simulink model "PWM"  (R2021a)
settings: Solver=FixedStepDiscrete  StartTime=0.0  StopTime=Inf  RelTol=1e-3  EnableMultiTasking=on
undefined symbols (not defined in the file or in its folder): A, ADCIN0, ADCIN1, ADCINA0, ADCINB0, bit, Compare, conversion, Count, DCAEVT1, DCAEVT1FILT, Digital, Down, edge, ended, Event, falling, Filtered, GPTRIP1SEL, GPTRIP2SEL, input, Module, of, resolution, rising, Single, start, the, Trip, TZ1, TZ2, Up, version, Zone
libraries: c2802xlib x9, c280xlib x2

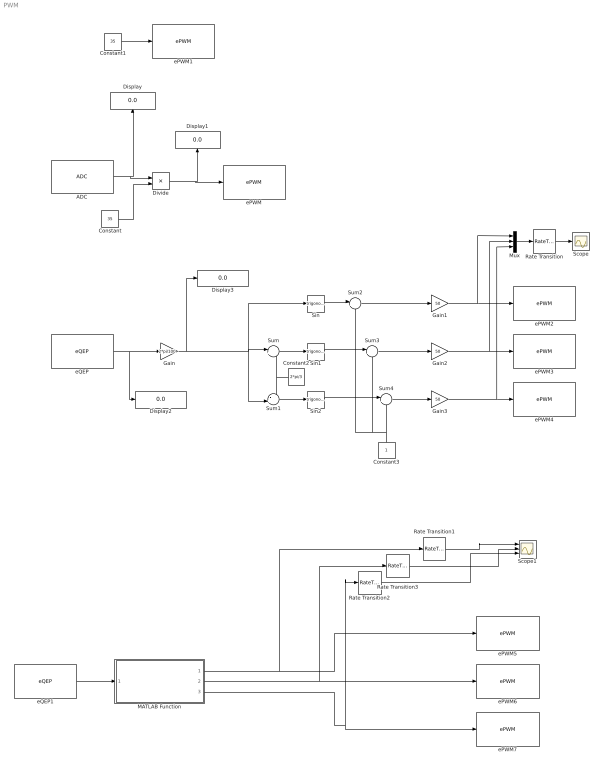
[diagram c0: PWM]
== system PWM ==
  ADC : c2802xlib/ADC  Commented=on  blkParamProc=C2000  ADCModule=1  samplingMode=Single sample mode  ADCResolution=12-bit (Single-ended input)  useSOC1=SOC0  useSOC2=SOC0_SOC1  SOCAcquisitionWindow=7  SOCTriggerSource=CPU0_TINT0n  SOCInterruptTrigger=No ADCINT  Ts=0.001  dType=uint16  postInterrupt=off  interruptSel=ADCINT1  ADCINTContinuous=off  endma=off  chdma=1  conv1=ADCINA6  conv2=ADCINA0 and ADCINB0  conv1_Type4=ADCIN0  conv2_Type4=ADCIN0 and ADCIN1
  Constant : Constant  Commented=on  Value=35
  Constant1 : Constant  Commented=on  Value=35
  Constant2 : Constant  Commented=on  Value=2*pi/3
  Constant3 : Constant  Commented=on
  Display{,1..3} (4 alike) : Display
  Divide : Product  Commented=on  Inputs=*/
  Gain : Gain  Commented=on  Gain=2*pi/100
  Gain1 : Gain  Commented=on  Gain=50
  Gain2 : Gain  Commented=on  Gain=50
  Gain3 : Gain  Commented=on  Gain=50
  MATLAB Function : MATLAB Function  TreatAsAtomicUnit=on
  Mux : Mux  Commented=on  Inputs=3
  Rate Transition : RateTransition  Commented=on
  Rate Transition1 : RateTransition
  Rate Transition2 : RateTransition
  Rate Transition3 : RateTransition
  Scope : Scope
  Scope1 : Scope  NumInputPorts=3
  Sin : Trigonometry  Commented=on
  Sin1 : Trigonometry  Commented=on
  Sin2 : Trigonometry  Commented=on
  Sum{,2..4} (4 alike) : Sum  Commented=on  Inputs=|++
  Sum1 : Sum  Commented=on  Inputs=-+|
  ePWM : c2802xlib/ePWM  Commented=on  PwmType=C2000  useModule=ePWM4  ePWMxLINKTBPRD=Not Linked  periodUnits=Seconds  timerSource=Specify via dialog  timerPeriod_clk=64000  timerPeriod_sec=0.0001  tbshadow=Counter equals to zero  countingMode=Up-Down  phaseActiveEnable=Disable  phaseDirection=Count down after sync  phaseActive=0  synchronizationEnable=off  dcaevt1Sync=off  dcbevt1Sync=off  synchronizationOption=Disable  perSynchronizationOption=Counter equals to period (CTR=PRD)  clockPrescale=1  HSclockPrescale=1  enswap=off  ePWMxAStatus=on  ePWMxAactionLogic1=Do nothing  ePWMxAactionLogic2=Do nothing  ePWMxAactionLogic3=Set  ePWMxAactionLogic4=Clear  ePWMxAactionLogic5=Do nothing  ePWMxAactionLogic6=Do nothing  ePWMxACSFenable=off  ePWMxACSFvalue=Forcing disable  ePWMxASFreload=Zero  ePWMxBStatus=off  ePWMxBactionLogic1=Set  ePWMxBactionLogic2=Clear  ePWMxBactionLogic3=Do nothing  ePWMxBactionLogic4=Do nothing  ePWMxBactionLogic5=Clear  ePWMxBactionLogic6=Set  ePWMxBCSFenable=off  ePWMxBCSFvalue=Forcing disable  ePWMxBSFreload=Zero  ePWNxBOutWay=off  ePWMxLINKCMPA=Not Linked  CMPAUnits=Percentages  CMPASource=Input port  CMPAValue_per=0  CMPAValue_clk=32000  enCMPAshadow=Counter equals to zero (CTR=Zero)  ePWMxLINKCMPB=Not Linked  CMPBUnits=Clock cycles  CMPBSource=Specify via dialog  CMPBValue_per=50  CMPBValue_clk=32000  enCMPBshadow=Counter equals to zero (CTR=Zero)  ePWMxLINKCMPC=Not Linked  CMPCUnits=Clock cycles  CMPCSource=Specify via dialog  CMPCValue_per=50  CMPCValue_clk=32000  enCMPCshadow=Counter equals to zero (CTR=Zero)  ePWMxLINKCMPD=Not Linked  CMPDUnits=Clock cycles  CMPDSource=Specify via dialog  CMPDValue_per=50  CMPDValue_clk=32000  enCMPDshadow=Counter equals to zero (CTR=Zero)  enableDBePWMxA=off  enableDBePWMxB=off  enhalfcycle=off  DBpolarity=Active high (AH)  DBedgeDelay=Positive  DBSource_ePWMxA=ePWMxA  DBSource_ePWMxB=ePWMxA  DBPeriodUnits=Clock cycles  DBperiodSource=Specify via dialog  REDperiod=0  FEDperiod=0  REDperiod_sec=0  FEDperiod_sec=0  LoadModeDBRED=Immediate without using shadow  LoadModeDBFED=Immediate without using shadow  adcstartModuleA=off  adcrequestEventA=First event  adcstartEventA=Counter equals to zero (CTR=Zero)  adcstartEventA_type2=Digital Compare Module A Event 1 start of conversion (DCAEVT1.soc)  adcstartModuleB=off  adcrequestEventB=First event  adcstartEventB=Counter equals to zero (CTR=Zero)  adcstartEventB_type2=Counter equals to zero (CTR=Zero)  intEn=off  intPrd=First event  intSel=Counter equals to zero (CTR=Zero)  intSel_type2=Counter equals to zero (CTR=Zero)  hrpe=off  enHRPWM=off  HRPWM_LoadMode=Counter equals to period (CTR=PRD)  HRPWM_CTLMode=Duty or Period control mode  HRPWM_EDGMode=Both edge  hrpeb=off  enHRPWMB=off  HRPWM_LoadModeB=Counter equals to zero (CTR=ZERO)  HRPWM_CTLModeB=Duty or Period control mode  HRPWM_EDGModeB=Both edge  enHRDBRED=off  enHRDBFED=off  enSFO=on  enautoconv=on  chopperEnable=off  chopperFrequency=1  chopperFirstwidth=1  chopperDuty=12.5%  tripZonesource=Specify via dialog  tzselOSHT1=off  tzselOSHT2=off  tzselOSHT3=off  tzselOSHDCAEV1=off  tzselOSHDCBEV1=off  tzselCBC1=off  tzselCBC2=off  tzselCBC3=off  tzselCBCDCAEV2=off  tzselCBCDCBEV2=off  tzselOSHT4=off  tzselOSHT5=off  tzselOSHT6=off  tzselCBC4=off  tzselCBC5=off  tzselCBC6=off  enTzOstIntr=off  enTzCbcIntr=off  enTzDCAEVT1Intr=off  enTzDCAEVT2Intr=off  enTzDCBEVT1Intr=off  enTzDCBEVT2Intr=off  ePWMxAforced=No action  ePWMxBforced=No action  DCAEVT1forced=No action  DCBEVT1forced=No action  DCAEVT2forced=No action  DCBEVT2forced=No action  dcah=Trip Zone 1 input (TZ1)  dcal=Trip Zone 1 input (TZ1)  dcbh=Trip Zone 1 input (TZ1)  dcbl=Trip Zone 1 input (TZ1)  dcah_type2=GPTRIP1SEL/(TZ1)  dcal_type2=GPTRIP2SEL/(TZ2)  dcbh_type2=GPTRIP1SEL/(TZ1)  dcbl_type2=GPTRIP2SEL/(TZ2)  gendcaevt1=Event disabled  gendcaevt2=Event disabled  gendcbevt1=Event disabled  gendcbevt2=Event disabled  dcaevt1src=DCAEVT1 with sync  dcaevt2src=DCAEVT2 with sync  dcbevt1src=DCBEVT1 with sync  dcbevt2src=DCBEVT2 with sync  pulsesel=Counter equals to zero (CTR=Zero)  blankinv=off  blankoffset=0  blankwidth=0  evsrcsel=Filtered version of DCAEVT1 (DCAEVT1FILT)  encape=off
  ePWM1 : c2802xlib/ePWM  Commented=on  PwmType=C2000  useModule=ePWM4  ePWMxLINKTBPRD=Not Linked  periodUnits=Seconds  timerSource=Specify via dialog  timerPeriod_clk=64000  timerPeriod_sec=0.0001  tbshadow=Counter equals to zero  countingMode=Up-Down  phaseActiveEnable=Disable  phaseDirection=Count down after sync  phaseActive=0  synchronizationEnable=off  dcaevt1Sync=off  dcbevt1Sync=off  synchronizationOption=Disable  perSynchronizationOption=Counter equals to period (CTR=PRD)  clockPrescale=1  HSclockPrescale=1  enswap=off  ePWMxAStatus=on  ePWMxAactionLogic1=Do nothing  ePWMxAactionLogic2=Do nothing  ePWMxAactionLogic3=Set  ePWMxAactionLogic4=Clear  ePWMxAactionLogic5=Do nothing  ePWMxAactionLogic6=Do nothing  ePWMxACSFenable=off  ePWMxACSFvalue=Forcing disable  ePWMxASFreload=Zero  ePWMxBStatus=off  ePWMxBactionLogic1=Set  ePWMxBactionLogic2=Clear  ePWMxBactionLogic3=Do nothing  ePWMxBactionLogic4=Do nothing  ePWMxBactionLogic5=Clear  ePWMxBactionLogic6=Set  ePWMxBCSFenable=off  ePWMxBCSFvalue=Forcing disable  ePWMxBSFreload=Zero  ePWNxBOutWay=off  ePWMxLINKCMPA=Not Linked  CMPAUnits=Percentages  CMPASource=Input port  CMPAValue_per=0  CMPAValue_clk=32000  enCMPAshadow=Counter equals to zero (CTR=Zero)  ePWMxLINKCMPB=Not Linked  CMPBUnits=Clock cycles  CMPBSource=Specify via dialog  CMPBValue_per=50  CMPBValue_clk=32000  enCMPBshadow=Counter equals to zero (CTR=Zero)  ePWMxLINKCMPC=Not Linked  CMPCUnits=Clock cycles  CMPCSource=Specify via dialog  CMPCValue_per=50  CMPCValue_clk=32000  enCMPCshadow=Counter equals to zero (CTR=Zero)  ePWMxLINKCMPD=Not Linked  CMPDUnits=Clock cycles  CMPDSource=Specify via dialog  CMPDValue_per=50  CMPDValue_clk=32000  enCMPDshadow=Counter equals to zero (CTR=Zero)  enableDBePWMxA=off  enableDBePWMxB=off  enhalfcycle=off  DBpolarity=Active high (AH)  DBedgeDelay=Positive  DBSource_ePWMxA=ePWMxA  DBSource_ePWMxB=ePWMxA  DBPeriodUnits=Clock cycles  DBperiodSource=Specify via dialog  REDperiod=0  FEDperiod=0  REDperiod_sec=0  FEDperiod_sec=0  LoadModeDBRED=Immediate without using shadow  LoadModeDBFED=Immediate without using shadow  adcstartModuleA=off  adcrequestEventA=First event  adcstartEventA=Counter equals to zero (CTR=Zero)  adcstartEventA_type2=Digital Compare Module A Event 1 start of conversion (DCAEVT1.soc)  adcstartModuleB=off  adcrequestEventB=First event  adcstartEventB=Counter equals to zero (CTR=Zero)  adcstartEventB_type2=Counter equals to zero (CTR=Zero)  intEn=off  intPrd=First event  intSel=Counter equals to zero (CTR=Zero)  intSel_type2=Counter equals to zero (CTR=Zero)  hrpe=off  enHRPWM=off  HRPWM_LoadMode=Counter equals to period (CTR=PRD)  HRPWM_CTLMode=Duty or Period control mode  HRPWM_EDGMode=Both edge  hrpeb=off  enHRPWMB=off  HRPWM_LoadModeB=Counter equals to zero (CTR=ZERO)  HRPWM_CTLModeB=Duty or Period control mode  HRPWM_EDGModeB=Both edge  enHRDBRED=off  enHRDBFED=off  enSFO=on  enautoconv=on  chopperEnable=off  chopperFrequency=1  chopperFirstwidth=1  chopperDuty=12.5%  tripZonesource=Specify via dialog  tzselOSHT1=off  tzselOSHT2=off  tzselOSHT3=off  tzselOSHDCAEV1=off  tzselOSHDCBEV1=off  tzselCBC1=off  tzselCBC2=off  tzselCBC3=off  tzselCBCDCAEV2=off  tzselCBCDCBEV2=off  tzselOSHT4=off  tzselOSHT5=off  tzselOSHT6=off  tzselCBC4=off  tzselCBC5=off  tzselCBC6=off  enTzOstIntr=off  enTzCbcIntr=off  enTzDCAEVT1Intr=off  enTzDCAEVT2Intr=off  enTzDCBEVT1Intr=off  enTzDCBEVT2Intr=off  ePWMxAforced=No action  ePWMxBforced=No action  DCAEVT1forced=No action  DCBEVT1forced=No action  DCAEVT2forced=No action  DCBEVT2forced=No action  dcah=Trip Zone 1 input (TZ1)  dcal=Trip Zone 1 input (TZ1)  dcbh=Trip Zone 1 input (TZ1)  dcbl=Trip Zone 1 input (TZ1)  dcah_type2=GPTRIP1SEL/(TZ1)  dcal_type2=GPTRIP2SEL/(TZ2)  dcbh_type2=GPTRIP1SEL/(TZ1)  dcbl_type2=GPTRIP2SEL/(TZ2)  gendcaevt1=Event disabled  gendcaevt2=Event disabled  gendcbevt1=Event disabled  gendcbevt2=Event disabled  dcaevt1src=DCAEVT1 with sync  dcaevt2src=DCAEVT2 with sync  dcbevt1src=DCBEVT1 with sync  dcbevt2src=DCBEVT2 with sync  pulsesel=Counter equals to zero (CTR=Zero)  blankinv=off  blankoffset=0  blankwidth=0  evsrcsel=Filtered version of DCAEVT1 (DCAEVT1FILT)  encape=off
  ePWM2 : c2802xlib/ePWM  Commented=on  PwmType=C2000  useModule=ePWM4  ePWMxLINKTBPRD=Not Linked  periodUnits=Seconds  timerSource=Specify via dialog  timerPeriod_clk=64000  timerPeriod_sec=0.0001  tbshadow=Counter equals to zero  countingMode=Up-Down  phaseActiveEnable=Disable  phaseDirection=Count down after sync  phaseActive=0  synchronizationEnable=off  dcaevt1Sync=off  dcbevt1Sync=off  synchronizationOption=Disable  perSynchronizationOption=Counter equals to period (CTR=PRD)  clockPrescale=1  HSclockPrescale=1  enswap=off  ePWMxAStatus=on  ePWMxAactionLogic1=Do nothing  ePWMxAactionLogic2=Do nothing  ePWMxAactionLogic3=Set  ePWMxAactionLogic4=Clear  ePWMxAactionLogic5=Do nothing  ePWMxAactionLogic6=Do nothing  ePWMxACSFenable=off  ePWMxACSFvalue=Forcing disable  ePWMxASFreload=Zero  ePWMxBStatus=off  ePWMxBactionLogic1=Set  ePWMxBactionLogic2=Clear  ePWMxBactionLogic3=Do nothing  ePWMxBactionLogic4=Do nothing  ePWMxBactionLogic5=Clear  ePWMxBactionLogic6=Set  ePWMxBCSFenable=off  ePWMxBCSFvalue=Forcing disable  ePWMxBSFreload=Zero  ePWNxBOutWay=off  ePWMxLINKCMPA=Not Linked  CMPAUnits=Percentages  CMPASource=Input port  CMPAValue_per=0  CMPAValue_clk=32000  enCMPAshadow=Counter equals to zero (CTR=Zero)  ePWMxLINKCMPB=Not Linked  CMPBUnits=Clock cycles  CMPBSource=Specify via dialog  CMPBValue_per=50  CMPBValue_clk=32000  enCMPBshadow=Counter equals to zero (CTR=Zero)  ePWMxLINKCMPC=Not Linked  CMPCUnits=Clock cycles  CMPCSource=Specify via dialog  CMPCValue_per=50  CMPCValue_clk=32000  enCMPCshadow=Counter equals to zero (CTR=Zero)  ePWMxLINKCMPD=Not Linked  CMPDUnits=Clock cycles  CMPDSource=Specify via dialog  CMPDValue_per=50  CMPDValue_clk=32000  enCMPDshadow=Counter equals to zero (CTR=Zero)  enableDBePWMxA=off  enableDBePWMxB=off  enhalfcycle=off  DBpolarity=Active high (AH)  DBedgeDelay=Positive  DBSource_ePWMxA=ePWMxA  DBSource_ePWMxB=ePWMxA  DBPeriodUnits=Clock cycles  DBperiodSource=Specify via dialog  REDperiod=0  FEDperiod=0  REDperiod_sec=0  FEDperiod_sec=0  LoadModeDBRED=Immediate without using shadow  LoadModeDBFED=Immediate without using shadow  adcstartModuleA=off  adcrequestEventA=First event  adcstartEventA=Counter equals to zero (CTR=Zero)  adcstartEventA_type2=Digital Compare Module A Event 1 start of conversion (DCAEVT1.soc)  adcstartModuleB=off  adcrequestEventB=First event  adcstartEventB=Counter equals to zero (CTR=Zero)  adcstartEventB_type2=Counter equals to zero (CTR=Zero)  intEn=off  intPrd=First event  intSel=Counter equals to zero (CTR=Zero)  intSel_type2=Counter equals to zero (CTR=Zero)  hrpe=off  enHRPWM=off  HRPWM_LoadMode=Counter equals to period (CTR=PRD)  HRPWM_CTLMode=Duty or Period control mode  HRPWM_EDGMode=Both edge  hrpeb=off  enHRPWMB=off  HRPWM_LoadModeB=Counter equals to zero (CTR=ZERO)  HRPWM_CTLModeB=Duty or Period control mode  HRPWM_EDGModeB=Both edge  enHRDBRED=off  enHRDBFED=off  enSFO=on  enautoconv=on  chopperEnable=off  chopperFrequency=1  chopperFirstwidth=1  chopperDuty=12.5%  tripZonesource=Specify via dialog  tzselOSHT1=off  tzselOSHT2=off  tzselOSHT3=off  tzselOSHDCAEV1=off  tzselOSHDCBEV1=off  tzselCBC1=off  tzselCBC2=off  tzselCBC3=off  tzselCBCDCAEV2=off  tzselCBCDCBEV2=off  tzselOSHT4=off  tzselOSHT5=off  tzselOSHT6=off  tzselCBC4=off  tzselCBC5=off  tzselCBC6=off  enTzOstIntr=off  enTzCbcIntr=off  enTzDCAEVT1Intr=off  enTzDCAEVT2Intr=off  enTzDCBEVT1Intr=off  enTzDCBEVT2Intr=off  ePWMxAforced=No action  ePWMxBforced=No action  DCAEVT1forced=No action  DCBEVT1forced=No action  DCAEVT2forced=No action  DCBEVT2forced=No action  dcah=Trip Zone 1 input (TZ1)  dcal=Trip Zone 1 input (TZ1)  dcbh=Trip Zone 1 input (TZ1)  dcbl=Trip Zone 1 input (TZ1)  dcah_type2=GPTRIP1SEL/(TZ1)  dcal_type2=GPTRIP2SEL/(TZ2)  dcbh_type2=GPTRIP1SEL/(TZ1)  dcbl_type2=GPTRIP2SEL/(TZ2)  gendcaevt1=Event disabled  gendcaevt2=Event disabled  gendcbevt1=Event disabled  gendcbevt2=Event disabled  dcaevt1src=DCAEVT1 with sync  dcaevt2src=DCAEVT2 with sync  dcbevt1src=DCBEVT1 with sync  dcbevt2src=DCBEVT2 with sync  pulsesel=Counter equals to zero (CTR=Zero)  blankinv=off  blankoffset=0  blankwidth=0  evsrcsel=Filtered version of DCAEVT1 (DCAEVT1FILT)  encape=off
  ePWM3 : c2802xlib/ePWM  Commented=on  PwmType=C2000  useModule=ePWM5  ePWMxLINKTBPRD=Not Linked  periodUnits=Seconds  timerSource=Specify via dialog  timerPeriod_clk=64000  timerPeriod_sec=0.0001  tbshadow=Counter equals to zero  countingMode=Up-Down  phaseActiveEnable=Disable  phaseDirection=Count down after sync  phaseActive=0  synchronizationEnable=off  dcaevt1Sync=off  dcbevt1Sync=off  synchronizationOption=Disable  perSynchronizationOption=Counter equals to period (CTR=PRD)  clockPrescale=1  HSclockPrescale=1  enswap=off  ePWMxAStatus=on  ePWMxAactionLogic1=Do nothing  ePWMxAactionLogic2=Do nothing  ePWMxAactionLogic3=Set  ePWMxAactionLogic4=Clear  ePWMxAactionLogic5=Do nothing  ePWMxAactionLogic6=Do nothing  ePWMxACSFenable=off  ePWMxACSFvalue=Forcing disable  ePWMxASFreload=Zero  ePWMxBStatus=off  ePWMxBactionLogic1=Set  ePWMxBactionLogic2=Clear  ePWMxBactionLogic3=Do nothing  ePWMxBactionLogic4=Do nothing  ePWMxBactionLogic5=Clear  ePWMxBactionLogic6=Set  ePWMxBCSFenable=off  ePWMxBCSFvalue=Forcing disable  ePWMxBSFreload=Zero  ePWNxBOutWay=off  ePWMxLINKCMPA=Not Linked  CMPAUnits=Percentages  CMPASource=Input port  CMPAValue_per=0  CMPAValue_clk=32000  enCMPAshadow=Counter equals to zero (CTR=Zero)  ePWMxLINKCMPB=Not Linked  CMPBUnits=Clock cycles  CMPBSource=Specify via dialog  CMPBValue_per=50  CMPBValue_clk=32000  enCMPBshadow=Counter equals to zero (CTR=Zero)  ePWMxLINKCMPC=Not Linked  CMPCUnits=Clock cycles  CMPCSource=Specify via dialog  CMPCValue_per=50  CMPCValue_clk=32000  enCMPCshadow=Counter equals to zero (CTR=Zero)  ePWMxLINKCMPD=Not Linked  CMPDUnits=Clock cycles  CMPDSource=Specify via dialog  CMPDValue_per=50  CMPDValue_clk=32000  enCMPDshadow=Counter equals to zero (CTR=Zero)  enableDBePWMxA=off  enableDBePWMxB=off  enhalfcycle=off  DBpolarity=Active high (AH)  DBedgeDelay=Positive  DBSource_ePWMxA=ePWMxA  DBSource_ePWMxB=ePWMxA  DBPeriodUnits=Clock cycles  DBperiodSource=Specify via dialog  REDperiod=0  FEDperiod=0  REDperiod_sec=0  FEDperiod_sec=0  LoadModeDBRED=Immediate without using shadow  LoadModeDBFED=Immediate without using shadow  adcstartModuleA=off  adcrequestEventA=First event  adcstartEventA=Counter equals to zero (CTR=Zero)  adcstartEventA_type2=Digital Compare Module A Event 1 start of conversion (DCAEVT1.soc)  adcstartModuleB=off  adcrequestEventB=First event  adcstartEventB=Counter equals to zero (CTR=Zero)  adcstartEventB_type2=Counter equals to zero (CTR=Zero)  intEn=off  intPrd=First event  intSel=Counter equals to zero (CTR=Zero)  intSel_type2=Counter equals to zero (CTR=Zero)  hrpe=off  enHRPWM=off  HRPWM_LoadMode=Counter equals to period (CTR=PRD)  HRPWM_CTLMode=Duty or Period control mode  HRPWM_EDGMode=Both edge  hrpeb=off  enHRPWMB=off  HRPWM_LoadModeB=Counter equals to zero (CTR=ZERO)  HRPWM_CTLModeB=Duty or Period control mode  HRPWM_EDGModeB=Both edge  enHRDBRED=off  enHRDBFED=off  enSFO=on  enautoconv=on  chopperEnable=off  chopperFrequency=1  chopperFirstwidth=1  chopperDuty=12.5%  tripZonesource=Specify via dialog  tzselOSHT1=off  tzselOSHT2=off  tzselOSHT3=off  tzselOSHDCAEV1=off  tzselOSHDCBEV1=off  tzselCBC1=off  tzselCBC2=off  tzselCBC3=off  tzselCBCDCAEV2=off  tzselCBCDCBEV2=off  tzselOSHT4=off  tzselOSHT5=off  tzselOSHT6=off  tzselCBC4=off  tzselCBC5=off  tzselCBC6=off  enTzOstIntr=off  enTzCbcIntr=off  enTzDCAEVT1Intr=off  enTzDCAEVT2Intr=off  enTzDCBEVT1Intr=off  enTzDCBEVT2Intr=off  ePWMxAforced=No action  ePWMxBforced=No action  DCAEVT1forced=No action  DCBEVT1forced=No action  DCAEVT2forced=No action  DCBEVT2forced=No action  dcah=Trip Zone 1 input (TZ1)  dcal=Trip Zone 1 input (TZ1)  dcbh=Trip Zone 1 input (TZ1)  dcbl=Trip Zone 1 input (TZ1)  dcah_type2=GPTRIP1SEL/(TZ1)  dcal_type2=GPTRIP2SEL/(TZ2)  dcbh_type2=GPTRIP1SEL/(TZ1)  dcbl_type2=GPTRIP2SEL/(TZ2)  gendcaevt1=Event disabled  gendcaevt2=Event disabled  gendcbevt1=Event disabled  gendcbevt2=Event disabled  dcaevt1src=DCAEVT1 with sync  dcaevt2src=DCAEVT2 with sync  dcbevt1src=DCBEVT1 with sync  dcbevt2src=DCBEVT2 with sync  pulsesel=Counter equals to zero (CTR=Zero)  blankinv=off  blankoffset=0  blankwidth=0  evsrcsel=Filtered version of DCAEVT1 (DCAEVT1FILT)  encape=off
  ePWM4 : c2802xlib/ePWM  Commented=on  PwmType=C2000  useModule=ePWM6  ePWMxLINKTBPRD=Not Linked  periodUnits=Seconds  timerSource=Specify via dialog  timerPeriod_clk=64000  timerPeriod_sec=0.0001  tbshadow=Counter equals to zero  countingMode=Up-Down  phaseActiveEnable=Disable  phaseDirection=Count down after sync  phaseActive=0  synchronizationEnable=off  dcaevt1Sync=off  dcbevt1Sync=off  synchronizationOption=Disable  perSynchronizationOption=Counter equals to period (CTR=PRD)  clockPrescale=1  HSclockPrescale=1  enswap=off  ePWMxAStatus=on  ePWMxAactionLogic1=Do nothing  ePWMxAactionLogic2=Do nothing  ePWMxAactionLogic3=Set  ePWMxAactionLogic4=Clear  ePWMxAactionLogic5=Do nothing  ePWMxAactionLogic6=Do nothing  ePWMxACSFenable=off  ePWMxACSFvalue=Forcing disable  ePWMxASFreload=Zero  ePWMxBStatus=off  ePWMxBactionLogic1=Set  ePWMxBactionLogic2=Clear  ePWMxBactionLogic3=Do nothing  ePWMxBactionLogic4=Do nothing  ePWMxBactionLogic5=Clear  ePWMxBactionLogic6=Set  ePWMxBCSFenable=off  ePWMxBCSFvalue=Forcing disable  ePWMxBSFreload=Zero  ePWNxBOutWay=off  ePWMxLINKCMPA=Not Linked  CMPAUnits=Percentages  CMPASource=Input port  CMPAValue_per=0  CMPAValue_clk=32000  enCMPAshadow=Counter equals to zero (CTR=Zero)  ePWMxLINKCMPB=Not Linked  CMPBUnits=Clock cycles  CMPBSource=Specify via dialog  CMPBValue_per=50  CMPBValue_clk=32000  enCMPBshadow=Counter equals to zero (CTR=Zero)  ePWMxLINKCMPC=Not Linked  CMPCUnits=Clock cycles  CMPCSource=Specify via dialog  CMPCValue_per=50  CMPCValue_clk=32000  enCMPCshadow=Counter equals to zero (CTR=Zero)  ePWMxLINKCMPD=Not Linked  CMPDUnits=Clock cycles  CMPDSource=Specify via dialog  CMPDValue_per=50  CMPDValue_clk=32000  enCMPDshadow=Counter equals to zero (CTR=Zero)  enableDBePWMxA=off  enableDBePWMxB=off  enhalfcycle=off  DBpolarity=Active high (AH)  DBedgeDelay=Positive  DBSource_ePWMxA=ePWMxA  DBSource_ePWMxB=ePWMxA  DBPeriodUnits=Clock cycles  DBperiodSource=Specify via dialog  REDperiod=0  FEDperiod=0  REDperiod_sec=0  FEDperiod_sec=0  LoadModeDBRED=Immediate without using shadow  LoadModeDBFED=Immediate without using shadow  adcstartModuleA=off  adcrequestEventA=First event  adcstartEventA=Counter equals to zero (CTR=Zero)  adcstartEventA_type2=Digital Compare Module A Event 1 start of conversion (DCAEVT1.soc)  adcstartModuleB=off  adcrequestEventB=First event  adcstartEventB=Counter equals to zero (CTR=Zero)  adcstartEventB_type2=Counter equals to zero (CTR=Zero)  intEn=off  intPrd=First event  intSel=Counter equals to zero (CTR=Zero)  intSel_type2=Counter equals to zero (CTR=Zero)  hrpe=off  enHRPWM=off  HRPWM_LoadMode=Counter equals to period (CTR=PRD)  HRPWM_CTLMode=Duty or Period control mode  HRPWM_EDGMode=Both edge  hrpeb=off  enHRPWMB=off  HRPWM_LoadModeB=Counter equals to zero (CTR=ZERO)  HRPWM_CTLModeB=Duty or Period control mode  HRPWM_EDGModeB=Both edge  enHRDBRED=off  enHRDBFED=off  enSFO=on  enautoconv=on  chopperEnable=off  chopperFrequency=1  chopperFirstwidth=1  chopperDuty=12.5%  tripZonesource=Specify via dialog  tzselOSHT1=off  tzselOSHT2=off  tzselOSHT3=off  tzselOSHDCAEV1=off  tzselOSHDCBEV1=off  tzselCBC1=off  tzselCBC2=off  tzselCBC3=off  tzselCBCDCAEV2=off  tzselCBCDCBEV2=off  tzselOSHT4=off  tzselOSHT5=off  tzselOSHT6=off  tzselCBC4=off  tzselCBC5=off  tzselCBC6=off  enTzOstIntr=off  enTzCbcIntr=off  enTzDCAEVT1Intr=off  enTzDCAEVT2Intr=off  enTzDCBEVT1Intr=off  enTzDCBEVT2Intr=off  ePWMxAforced=No action  ePWMxBforced=No action  DCAEVT1forced=No action  DCBEVT1forced=No action  DCAEVT2forced=No action  DCBEVT2forced=No action  dcah=Trip Zone 1 input (TZ1)  dcal=Trip Zone 1 input (TZ1)  dcbh=Trip Zone 1 input (TZ1)  dcbl=Trip Zone 1 input (TZ1)  dcah_type2=GPTRIP1SEL/(TZ1)  dcal_type2=GPTRIP2SEL/(TZ2)  dcbh_type2=GPTRIP1SEL/(TZ1)  dcbl_type2=GPTRIP2SEL/(TZ2)  gendcaevt1=Event disabled  gendcaevt2=Event disabled  gendcbevt1=Event disabled  gendcbevt2=Event disabled  dcaevt1src=DCAEVT1 with sync  dcaevt2src=DCAEVT2 with sync  dcbevt1src=DCBEVT1 with sync  dcbevt2src=DCBEVT2 with sync  pulsesel=Counter equals to zero (CTR=Zero)  blankinv=off  blankoffset=0  blankwidth=0  evsrcsel=Filtered version of DCAEVT1 (DCAEVT1FILT)  encape=off
  ePWM5 : c2802xlib/ePWM  PwmType=C2000  useModule=ePWM4  ePWMxLINKTBPRD=Not Linked  periodUnits=Seconds  timerSource=Specify via dialog  timerPeriod_clk=64000  timerPeriod_sec=0.0001  tbshadow=Counter equals to zero  countingMode=Up-Down  phaseActiveEnable=Disable  phaseDirection=Count down after sync  phaseActive=0  synchronizationEnable=off  dcaevt1Sync=off  dcbevt1Sync=off  synchronizationOption=Disable  perSynchronizationOption=Counter equals to period (CTR=PRD)  clockPrescale=1  HSclockPrescale=1  enswap=off  ePWMxAStatus=on  ePWMxAactionLogic1=Do nothing  ePWMxAactionLogic2=Do nothing  ePWMxAactionLogic3=Set  ePWMxAactionLogic4=Clear  ePWMxAactionLogic5=Do nothing  ePWMxAactionLogic6=Do nothing  ePWMxACSFenable=off  ePWMxACSFvalue=Forcing disable  ePWMxASFreload=Zero  ePWMxBStatus=off  ePWMxBactionLogic1=Set  ePWMxBactionLogic2=Clear  ePWMxBactionLogic3=Do nothing  ePWMxBactionLogic4=Do nothing  ePWMxBactionLogic5=Clear  ePWMxBactionLogic6=Set  ePWMxBCSFenable=off  ePWMxBCSFvalue=Forcing disable  ePWMxBSFreload=Zero  ePWNxBOutWay=off  ePWMxLINKCMPA=Not Linked  CMPAUnits=Percentages  CMPASource=Input port  CMPAValue_per=0  CMPAValue_clk=32000  enCMPAshadow=Counter equals to zero (CTR=Zero)  ePWMxLINKCMPB=Not Linked  CMPBUnits=Clock cycles  CMPBSource=Specify via dialog  CMPBValue_per=50  CMPBValue_clk=32000  enCMPBshadow=Counter equals to zero (CTR=Zero)  ePWMxLINKCMPC=Not Linked  CMPCUnits=Clock cycles  CMPCSource=Specify via dialog  CMPCValue_per=50  CMPCValue_clk=32000  enCMPCshadow=Counter equals to zero (CTR=Zero)  ePWMxLINKCMPD=Not Linked  CMPDUnits=Clock cycles  CMPDSource=Specify via dialog  CMPDValue_per=50  CMPDValue_clk=32000  enCMPDshadow=Counter equals to zero (CTR=Zero)  enableDBePWMxA=off  enableDBePWMxB=off  enhalfcycle=off  DBpolarity=Active high (AH)  DBedgeDelay=Positive  DBSource_ePWMxA=ePWMxA  DBSource_ePWMxB=ePWMxA  DBPeriodUnits=Clock cycles  DBperiodSource=Specify via dialog  REDperiod=0  FEDperiod=0  REDperiod_sec=0  FEDperiod_sec=0  LoadModeDBRED=Immediate without using shadow  LoadModeDBFED=Immediate without using shadow  adcstartModuleA=off  adcrequestEventA=First event  adcstartEventA=Counter equals to zero (CTR=Zero)  adcstartEventA_type2=Digital Compare Module A Event 1 start of conversion (DCAEVT1.soc)  adcstartModuleB=off  adcrequestEventB=First event  adcstartEventB=Counter equals to zero (CTR=Zero)  adcstartEventB_type2=Counter equals to zero (CTR=Zero)  intEn=off  intPrd=First event  intSel=Counter equals to zero (CTR=Zero)  intSel_type2=Counter equals to zero (CTR=Zero)  hrpe=off  enHRPWM=off  HRPWM_LoadMode=Counter equals to period (CTR=PRD)  HRPWM_CTLMode=Duty or Period control mode  HRPWM_EDGMode=Both edge  hrpeb=off  enHRPWMB=off  HRPWM_LoadModeB=Counter equals to zero (CTR=ZERO)  HRPWM_CTLModeB=Duty or Period control mode  HRPWM_EDGModeB=Both edge  enHRDBRED=off  enHRDBFED=off  enSFO=on  enautoconv=on  chopperEnable=off  chopperFrequency=1  chopperFirstwidth=1  chopperDuty=12.5%  tripZonesource=Specify via dialog  tzselOSHT1=off  tzselOSHT2=off  tzselOSHT3=off  tzselOSHDCAEV1=off  tzselOSHDCBEV1=off  tzselCBC1=off  tzselCBC2=off  tzselCBC3=off  tzselCBCDCAEV2=off  tzselCBCDCBEV2=off  tzselOSHT4=off  tzselOSHT5=off  tzselOSHT6=off  tzselCBC4=off  tzselCBC5=off  tzselCBC6=off  enTzOstIntr=off  enTzCbcIntr=off  enTzDCAEVT1Intr=off  enTzDCAEVT2Intr=off  enTzDCBEVT1Intr=off  enTzDCBEVT2Intr=off  ePWMxAforced=No action  ePWMxBforced=No action  DCAEVT1forced=No action  DCBEVT1forced=No action  DCAEVT2forced=No action  DCBEVT2forced=No action  dcah=Trip Zone 1 input (TZ1)  dcal=Trip Zone 1 input (TZ1)  dcbh=Trip Zone 1 input (TZ1)  dcbl=Trip Zone 1 input (TZ1)  dcah_type2=GPTRIP1SEL/(TZ1)  dcal_type2=GPTRIP2SEL/(TZ2)  dcbh_type2=GPTRIP1SEL/(TZ1)  dcbl_type2=GPTRIP2SEL/(TZ2)  gendcaevt1=Event disabled  gendcaevt2=Event disabled  gendcbevt1=Event disabled  gendcbevt2=Event disabled  dcaevt1src=DCAEVT1 with sync  dcaevt2src=DCAEVT2 with sync  dcbevt1src=DCBEVT1 with sync  dcbevt2src=DCBEVT2 with sync  pulsesel=Counter equals to zero (CTR=Zero)  blankinv=off  blankoffset=0  blankwidth=0  evsrcsel=Filtered version of DCAEVT1 (DCAEVT1FILT)  encape=off
  ePWM6 : c2802xlib/ePWM  PwmType=C2000  useModule=ePWM5  ePWMxLINKTBPRD=Not Linked  periodUnits=Seconds  timerSource=Specify via dialog  timerPeriod_clk=64000  timerPeriod_sec=0.0001  tbshadow=Counter equals to zero  countingMode=Up-Down  phaseActiveEnable=Disable  phaseDirection=Count down after sync  phaseActive=0  synchronizationEnable=off  dcaevt1Sync=off  dcbevt1Sync=off  synchronizationOption=Disable  perSynchronizationOption=Counter equals to period (CTR=PRD)  clockPrescale=1  HSclockPrescale=1  enswap=off  ePWMxAStatus=on  ePWMxAactionLogic1=Do nothing  ePWMxAactionLogic2=Do nothing  ePWMxAactionLogic3=Set  ePWMxAactionLogic4=Clear  ePWMxAactionLogic5=Do nothing  ePWMxAactionLogic6=Do nothing  ePWMxACSFenable=off  ePWMxACSFvalue=Forcing disable  ePWMxASFreload=Zero  ePWMxBStatus=off  ePWMxBactionLogic1=Set  ePWMxBactionLogic2=Clear  ePWMxBactionLogic3=Do nothing  ePWMxBactionLogic4=Do nothing  ePWMxBactionLogic5=Clear  ePWMxBactionLogic6=Set  ePWMxBCSFenable=off  ePWMxBCSFvalue=Forcing disable  ePWMxBSFreload=Zero  ePWNxBOutWay=off  ePWMxLINKCMPA=Not Linked  CMPAUnits=Percentages  CMPASource=Input port  CMPAValue_per=0  CMPAValue_clk=32000  enCMPAshadow=Counter equals to zero (CTR=Zero)  ePWMxLINKCMPB=Not Linked  CMPBUnits=Clock cycles  CMPBSource=Specify via dialog  CMPBValue_per=50  CMPBValue_clk=32000  enCMPBshadow=Counter equals to zero (CTR=Zero)  ePWMxLINKCMPC=Not Linked  CMPCUnits=Clock cycles  CMPCSource=Specify via dialog  CMPCValue_per=50  CMPCValue_clk=32000  enCMPCshadow=Counter equals to zero (CTR=Zero)  ePWMxLINKCMPD=Not Linked  CMPDUnits=Clock cycles  CMPDSource=Specify via dialog  CMPDValue_per=50  CMPDValue_clk=32000  enCMPDshadow=Counter equals to zero (CTR=Zero)  enableDBePWMxA=off  enableDBePWMxB=off  enhalfcycle=off  DBpolarity=Active high (AH)  DBedgeDelay=Positive  DBSource_ePWMxA=ePWMxA  DBSource_ePWMxB=ePWMxA  DBPeriodUnits=Clock cycles  DBperiodSource=Specify via dialog  REDperiod=0  FEDperiod=0  REDperiod_sec=0  FEDperiod_sec=0  LoadModeDBRED=Immediate without using shadow  LoadModeDBFED=Immediate without using shadow  adcstartModuleA=off  adcrequestEventA=First event  adcstartEventA=Counter equals to zero (CTR=Zero)  adcstartEventA_type2=Digital Compare Module A Event 1 start of conversion (DCAEVT1.soc)  adcstartModuleB=off  adcrequestEventB=First event  adcstartEventB=Counter equals to zero (CTR=Zero)  adcstartEventB_type2=Counter equals to zero (CTR=Zero)  intEn=off  intPrd=First event  intSel=Counter equals to zero (CTR=Zero)  intSel_type2=Counter equals to zero (CTR=Zero)  hrpe=off  enHRPWM=off  HRPWM_LoadMode=Counter equals to period (CTR=PRD)  HRPWM_CTLMode=Duty or Period control mode  HRPWM_EDGMode=Both edge  hrpeb=off  enHRPWMB=off  HRPWM_LoadModeB=Counter equals to zero (CTR=ZERO)  HRPWM_CTLModeB=Duty or Period control mode  HRPWM_EDGModeB=Both edge  enHRDBRED=off  enHRDBFED=off  enSFO=on  enautoconv=on  chopperEnable=off  chopperFrequency=1  chopperFirstwidth=1  chopperDuty=12.5%  tripZonesource=Specify via dialog  tzselOSHT1=off  tzselOSHT2=off  tzselOSHT3=off  tzselOSHDCAEV1=off  tzselOSHDCBEV1=off  tzselCBC1=off  tzselCBC2=off  tzselCBC3=off  tzselCBCDCAEV2=off  tzselCBCDCBEV2=off  tzselOSHT4=off  tzselOSHT5=off  tzselOSHT6=off  tzselCBC4=off  tzselCBC5=off  tzselCBC6=off  enTzOstIntr=off  enTzCbcIntr=off  enTzDCAEVT1Intr=off  enTzDCAEVT2Intr=off  enTzDCBEVT1Intr=off  enTzDCBEVT2Intr=off  ePWMxAforced=No action  ePWMxBforced=No action  DCAEVT1forced=No action  DCBEVT1forced=No action  DCAEVT2forced=No action  DCBEVT2forced=No action  dcah=Trip Zone 1 input (TZ1)  dcal=Trip Zone 1 input (TZ1)  dcbh=Trip Zone 1 input (TZ1)  dcbl=Trip Zone 1 input (TZ1)  dcah_type2=GPTRIP1SEL/(TZ1)  dcal_type2=GPTRIP2SEL/(TZ2)  dcbh_type2=GPTRIP1SEL/(TZ1)  dcbl_type2=GPTRIP2SEL/(TZ2)  gendcaevt1=Event disabled  gendcaevt2=Event disabled  gendcbevt1=Event disabled  gendcbevt2=Event disabled  dcaevt1src=DCAEVT1 with sync  dcaevt2src=DCAEVT2 with sync  dcbevt1src=DCBEVT1 with sync  dcbevt2src=DCBEVT2 with sync  pulsesel=Counter equals to zero (CTR=Zero)  blankinv=off  blankoffset=0  blankwidth=0  evsrcsel=Filtered version of DCAEVT1 (DCAEVT1FILT)  encape=off
  ePWM7 : c2802xlib/ePWM  PwmType=C2000  useModule=ePWM6  ePWMxLINKTBPRD=Not Linked  periodUnits=Seconds  timerSource=Specify via dialog  timerPeriod_clk=64000  timerPeriod_sec=0.0001  tbshadow=Counter equals to zero  countingMode=Up-Down  phaseActiveEnable=Disable  phaseDirection=Count down after sync  phaseActive=0  synchronizationEnable=off  dcaevt1Sync=off  dcbevt1Sync=off  synchronizationOption=Disable  perSynchronizationOption=Counter equals to period (CTR=PRD)  clockPrescale=1  HSclockPrescale=1  enswap=off  ePWMxAStatus=on  ePWMxAactionLogic1=Do nothing  ePWMxAactionLogic2=Do nothing  ePWMxAactionLogic3=Set  ePWMxAactionLogic4=Clear  ePWMxAactionLogic5=Do nothing  ePWMxAactionLogic6=Do nothing  ePWMxACSFenable=off  ePWMxACSFvalue=Forcing disable  ePWMxASFreload=Zero  ePWMxBStatus=off  ePWMxBactionLogic1=Set  ePWMxBactionLogic2=Clear  ePWMxBactionLogic3=Do nothing  ePWMxBactionLogic4=Do nothing  ePWMxBactionLogic5=Clear  ePWMxBactionLogic6=Set  ePWMxBCSFenable=off  ePWMxBCSFvalue=Forcing disable  ePWMxBSFreload=Zero  ePWNxBOutWay=off  ePWMxLINKCMPA=Not Linked  CMPAUnits=Percentages  CMPASource=Input port  CMPAValue_per=0  CMPAValue_clk=32000  enCMPAshadow=Counter equals to zero (CTR=Zero)  ePWMxLINKCMPB=Not Linked  CMPBUnits=Clock cycles  CMPBSource=Specify via dialog  CMPBValue_per=50  CMPBValue_clk=32000  enCMPBshadow=Counter equals to zero (CTR=Zero)  ePWMxLINKCMPC=Not Linked  CMPCUnits=Clock cycles  CMPCSource=Specify via dialog  CMPCValue_per=50  CMPCValue_clk=32000  enCMPCshadow=Counter equals to zero (CTR=Zero)  ePWMxLINKCMPD=Not Linked  CMPDUnits=Clock cycles  CMPDSource=Specify via dialog  CMPDValue_per=50  CMPDValue_clk=32000  enCMPDshadow=Counter equals to zero (CTR=Zero)  enableDBePWMxA=off  enableDBePWMxB=off  enhalfcycle=off  DBpolarity=Active high (AH)  DBedgeDelay=Positive  DBSource_ePWMxA=ePWMxA  DBSource_ePWMxB=ePWMxA  DBPeriodUnits=Clock cycles  DBperiodSource=Specify via dialog  REDperiod=0  FEDperiod=0  REDperiod_sec=0  FEDperiod_sec=0  LoadModeDBRED=Immediate without using shadow  LoadModeDBFED=Immediate without using shadow  adcstartModuleA=off  adcrequestEventA=First event  adcstartEventA=Counter equals to zero (CTR=Zero)  adcstartEventA_type2=Digital Compare Module A Event 1 start of conversion (DCAEVT1.soc)  adcstartModuleB=off  adcrequestEventB=First event  adcstartEventB=Counter equals to zero (CTR=Zero)  adcstartEventB_type2=Counter equals to zero (CTR=Zero)  intEn=off  intPrd=First event  intSel=Counter equals to zero (CTR=Zero)  intSel_type2=Counter equals to zero (CTR=Zero)  hrpe=off  enHRPWM=off  HRPWM_LoadMode=Counter equals to period (CTR=PRD)  HRPWM_CTLMode=Duty or Period control mode  HRPWM_EDGMode=Both edge  hrpeb=off  enHRPWMB=off  HRPWM_LoadModeB=Counter equals to zero (CTR=ZERO)  HRPWM_CTLModeB=Duty or Period control mode  HRPWM_EDGModeB=Both edge  enHRDBRED=off  enHRDBFED=off  enSFO=on  enautoconv=on  chopperEnable=off  chopperFrequency=1  chopperFirstwidth=1  chopperDuty=12.5%  tripZonesource=Specify via dialog  tzselOSHT1=off  tzselOSHT2=off  tzselOSHT3=off  tzselOSHDCAEV1=off  tzselOSHDCBEV1=off  tzselCBC1=off  tzselCBC2=off  tzselCBC3=off  tzselCBCDCAEV2=off  tzselCBCDCBEV2=off  tzselOSHT4=off  tzselOSHT5=off  tzselOSHT6=off  tzselCBC4=off  tzselCBC5=off  tzselCBC6=off  enTzOstIntr=off  enTzCbcIntr=off  enTzDCAEVT1Intr=off  enTzDCAEVT2Intr=off  enTzDCBEVT1Intr=off  enTzDCBEVT2Intr=off  ePWMxAforced=No action  ePWMxBforced=No action  DCAEVT1forced=No action  DCBEVT1forced=No action  DCAEVT2forced=No action  DCBEVT2forced=No action  dcah=Trip Zone 1 input (TZ1)  dcal=Trip Zone 1 input (TZ1)  dcbh=Trip Zone 1 input (TZ1)  dcbl=Trip Zone 1 input (TZ1)  dcah_type2=GPTRIP1SEL/(TZ1)  dcal_type2=GPTRIP2SEL/(TZ2)  dcbh_type2=GPTRIP1SEL/(TZ1)  dcbl_type2=GPTRIP2SEL/(TZ2)  gendcaevt1=Event disabled  gendcaevt2=Event disabled  gendcbevt1=Event disabled  gendcbevt2=Event disabled  dcaevt1src=DCAEVT1 with sync  dcaevt2src=DCAEVT2 with sync  dcbevt1src=DCBEVT1 with sync  dcbevt2src=DCBEVT2 with sync  pulsesel=Counter equals to zero (CTR=Zero)  blankinv=off  blankoffset=0  blankwidth=0  evsrcsel=Filtered version of DCAEVT1 (DCAEVT1FILT)  encape=off
  eQEP : c280xlib/eQEP  Commented=on  useModule=eQEP2  pcInputmode=Quadrature-count  externalClockrate=2x resolution: Count the rising/falling edge  swapPolarityselection=Clockwise  qdfOutputport=off  qapPolarityselection=off  qbpPolarityselection=off  qipPolarityselection=off  qspPolarityselection=off  igatePolarityselection=off  sampleTime=0.0001  pcOutputport=on  pcMaximumvalue=100  indexInitializationcheck=off  indexInitializationevent=Rising edge  strobeInitializationcheck=off  strobeInitializationevent=Rising edge  softwareInitializationcheck=off  softwareInitializationsource=Set to init value at start up  softwareInitializationmode=on  pcInitialvalue=2147483648  pcResetmode=Reset on the maximum position  ieloutputport=off  indexEventlatch=Rising edge  seloutputport=off  strobeEventlatch=Rising edge  pcefOutputport=off  enableEqepcapture=off  qctmrOutputport=off  qcprdOutputport=off  captureTimerprescaler=128  upEventprescaler=128  overflowErrorflag=off  directionErrorflag=off  captureTimerposition=On position counter read  unitTimerperiod=100000000  captureTimerlatch=off  capturePeriodlatch=off  positionCounterlatch=off  soenPolarityselection=off  spselPolarityselection=Index pin is used for sync output  compareValuesource=Specify via dialog  shadowMode=Load on QPOSCNT=0  compareValue=4294967295  syncOutputwidth=1  polaritySyncoutput=Active high  watchdogEnable=off  watchdogTimer=65535  outport1Datatype=auto  outport2Datatype=auto  outport3Datatype=auto  outport4Datatype=auto  outport5Datatype=auto  outport6Datatype=auto  outport7Datatype=auto  outport8Datatype=auto  outport9Datatype=auto  outport10Datatype=auto  outport11Datatype=auto  outport12Datatype=auto  eqepinterrupt_pce=off  eqepinterrupt_qpe=off  eqepinterrupt_qdc=off  eqepinterrupt_wto=off  eqepinterrupt_pcu=off  eqepinterrupt_pco=off  eqepinterrupt_pcr=off  eqepinterrupt_pcm=off  eqepinterrupt_sel=off  eqepinterrupt_iel=off  eqepinterrupt_uto=off  pheOutputport=off  watchdogOutputport=off  outport13Datatype=auto  outport14Datatype=auto
  eQEP1 : c280xlib/eQEP  useModule=eQEP2  pcInputmode=Quadrature-count  externalClockrate=2x resolution: Count the rising/falling edge  swapPolarityselection=Clockwise  qdfOutputport=off  qapPolarityselection=off  qbpPolarityselection=off  qipPolarityselection=off  qspPolarityselection=off  igatePolarityselection=off  sampleTime=0.001  pcOutputport=on  pcMaximumvalue=100  indexInitializationcheck=off  indexInitializationevent=Rising edge  strobeInitializationcheck=off  strobeInitializationevent=Rising edge  softwareInitializationcheck=off  softwareInitializationsource=Set to init value at start up  softwareInitializationmode=on  pcInitialvalue=2147483648  pcResetmode=Reset on the maximum position  ieloutputport=off  indexEventlatch=Rising edge  seloutputport=off  strobeEventlatch=Rising edge  pcefOutputport=off  enableEqepcapture=off  qctmrOutputport=off  qcprdOutputport=off  captureTimerprescaler=128  upEventprescaler=128  overflowErrorflag=off  directionErrorflag=off  captureTimerposition=On position counter read  unitTimerperiod=100000000  captureTimerlatch=off  capturePeriodlatch=off  positionCounterlatch=off  soenPolarityselection=off  spselPolarityselection=Index pin is used for sync output  compareValuesource=Specify via dialog  shadowMode=Load on QPOSCNT=0  compareValue=4294967295  syncOutputwidth=1  polaritySyncoutput=Active high  watchdogEnable=off  watchdogTimer=65535  outport1Datatype=auto  outport2Datatype=auto  outport3Datatype=auto  outport4Datatype=auto  outport5Datatype=auto  outport6Datatype=auto  outport7Datatype=auto  outport8Datatype=auto  outport9Datatype=auto  outport10Datatype=auto  outport11Datatype=auto  outport12Datatype=auto  eqepinterrupt_pce=off  eqepinterrupt_qpe=off  eqepinterrupt_qdc=off  eqepinterrupt_wto=off  eqepinterrupt_pcu=off  eqepinterrupt_pco=off  eqepinterrupt_pcr=off  eqepinterrupt_pcm=off  eqepinterrupt_sel=off  eqepinterrupt_iel=off  eqepinterrupt_uto=off  pheOutputport=off  watchdogOutputport=off  outport13Datatype=auto  outport14Datatype=auto
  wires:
  Divide/1 -> Display1/1, ePWM/1
  Constant/1 -> Divide/2
  ADC/1 -> Divide/1, Display/1
  Constant1/1 -> ePWM1/1
  eQEP/1 -> Gain/1, Display2/1
  Sum1/1 -> Sin2/1
  Sum/1 -> Sin1/1
  Gain/1 -> Sum1/2, Sin/1, Sum/1, Display3/1
  Constant2/1 -> Sum1/1, Sum/2
  Constant3/1 -> Sum2/2, Sum3/2, Sum4/2
  Sin2/1 -> Sum4/1
  Sin1/1 -> Sum3/1
  Sin/1 -> Sum2/1
  Gain1/1 -> Mux/1, ePWM2/1
  Gain2/1 -> Mux/2, ePWM3/1
  Gain3/1 -> Mux/3, ePWM4/1
  Sum4/1 -> Gain3/1
  Sum3/1 -> Gain2/1
  Sum2/1 -> Gain1/1
  Mux/1 -> Rate Transition/1
  Rate Transition/1 -> Scope/1
  eQEP1/1 -> MATLAB Function/1(pos)
  MATLAB Function/2(pwm2) -> Rate Transition3/1, ePWM6/1
  MATLAB Function/1(pwm1) -> Rate Transition1/1, ePWM5/1
  MATLAB Function/3(pwm3) -> Rate Transition2/1, ePWM7/1
  Rate Transition1/1 -> Scope1/1
  Rate Transition2/1 -> Scope1/3
  Rate Transition3/1 -> Scope1/2

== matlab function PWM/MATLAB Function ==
function [pwm1,pwm2,pwm3] = fcn(pos)
%#codegen

angle = pos *2*pi/100

pwm1 = (sin(angle)+1)*50;
pwm2 = (sin(angle+2*pi/3)+1)*50
pwm3 = (sin(angle-2*pi/3)+1)*50
